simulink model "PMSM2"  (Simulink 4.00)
settings: Solver=ode23  StartTime=-eps  StopTime=2  FixedStep=0.000001  RelTol=1e-3
undefined symbols (not defined in the file or in its folder): J, Lsx, Lsy, p, Psim, Rs, sfunxy, Ts, Udc

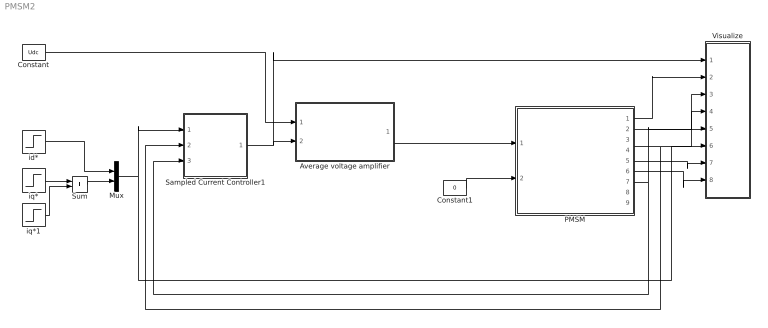
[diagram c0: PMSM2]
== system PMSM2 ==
  Average voltage amplifier : Subsystem
  Constant : Constant  Value=Udc
  Constant1 : Constant  Value=0
  Mux : Mux  Inputs=2
  PMSM : Subsystem  mask{Psim=Psim, p=p, Rs=Rs, isy=[0 1], psisy=[0 Lsy], isx=[0 1], psisx=[0 Lsx], J=J}
      mask prompts: p "Number of poles"; Rs "Stator resistance"; isy "y-axis current vector"; psisy "y-axis flux vector"; isx "x-axis current vector"; psisx "x-axis flux vector"; J "Inertia"
  Sampled Current Controller1 : Subsystem  mask{R=Rs, Lx=Lsx, Ly=Lsy, Kp=[(Lsx/Ts+Rs/2) (Lsy/Ts+Rs/2)]', Ti=[(Lsx/Rs+Ts/2) (Lsy/Rs+Ts/2)]', Ts=Ts, Umax=Udc, Umin=-Udc, SlowFast=Fast computer}
      mask prompts: R "Load resistance"; Lx "x-axis load inductance"; Ly "y-axis load inductance"; Kp "Controller gain"; Ti "Integral Time Constant"; Ts "Sampling time [s]"; Umax "Max output signal"; Umin "Min output signal"; SlowFast "Controller type"
  Sum : Sum  Inputs=++  SaturateOnIntegerOverflow=on
  Visualize : Subsystem
  id* : Step  Time=0.0105  Before=0  After=0  SampleTime=0
  iq* : Step  Time=0.0055  Before=0  After=10  SampleTime=0
  iq*1 : Step  Time=0.05  Before=0  After=0  SampleTime=0
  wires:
  Average voltage amplifier/1(vabc) -> PMSM/1(vabc)
  Sampled Current Controller1/1(u*) -> Visualize/1(u*), Average voltage amplifier/2(uabc*)
  Constant/1 -> Average voltage amplifier/1(Udc)
  id*/1 -> Mux/1
  Mux/1 -> Visualize/6(i*dq), Sampled Current Controller1/1(Ref_dq)
  PMSM/7(theta_el) -> Visualize/5(theta), Sampled Current Controller1/3(thetaR)
  Constant1/1 -> PMSM/2(Tl)
  PMSM/1(uabc) -> Visualize/2("u ")
  PMSM/4(is) -> Visualize/4(i), Sampled Current Controller1/2(Act_ab)
  PMSM/2(exy) -> Visualize/3(e)
  PMSM/5(T_mech) -> Visualize/7(Tmech)
  PMSM/6(w_mech) -> Visualize/8(wmech)
  iq*/1 -> Sum/1
  iq*1/1 -> Sum/2
  Sum/1 -> Mux/2

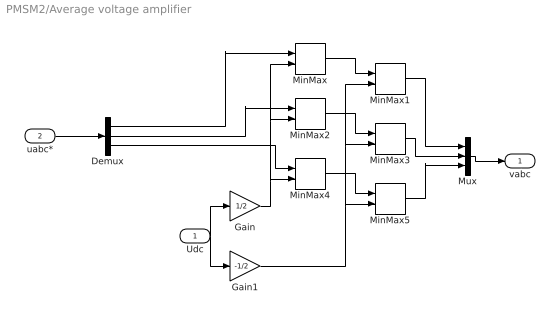
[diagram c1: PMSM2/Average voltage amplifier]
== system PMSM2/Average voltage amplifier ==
  Udc : Inport  Port=1  LatchInput=off
  uabc* : Inport  Port=2  LatchInput=off
  Demux : Demux  Outputs=3  BusSelectionMode=off
  Gain : Gain  Gain=1/2  Multiplication=Element-wise(K.*u)  SaturateOnIntegerOverflow=on
  Gain1 : Gain  Gain=-1/2  Multiplication=Element-wise(K.*u)  SaturateOnIntegerOverflow=on
  MinMax : MinMax  Function=min  Inputs=2
  MinMax1 : MinMax  Function=max  Inputs=2
  MinMax2 : MinMax  Function=min  Inputs=2
  MinMax3 : MinMax  Function=max  Inputs=2
  MinMax4 : MinMax  Function=min  Inputs=2
  MinMax5 : MinMax  Function=max  Inputs=2
  Mux : Mux  Inputs=3
  vabc : Outport  Port=1  InitialOutput=0
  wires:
  MinMax/1 -> MinMax1/1
  Udc/1 -> Gain/1, Gain1/1
  Gain/1 -> MinMax/2, MinMax2/2, MinMax4/2
  Gain1/1 -> MinMax1/2, MinMax3/2, MinMax5/2
  MinMax2/1 -> MinMax3/1
  MinMax4/1 -> MinMax5/1
  uabc*/1 -> Demux/1
  Demux/1 -> MinMax/1
  Demux/2 -> MinMax2/1
  Demux/3 -> MinMax4/1
  MinMax1/1 -> Mux/1
  MinMax3/1 -> Mux/2
  MinMax5/1 -> Mux/3
  Mux/1 -> vabc/1

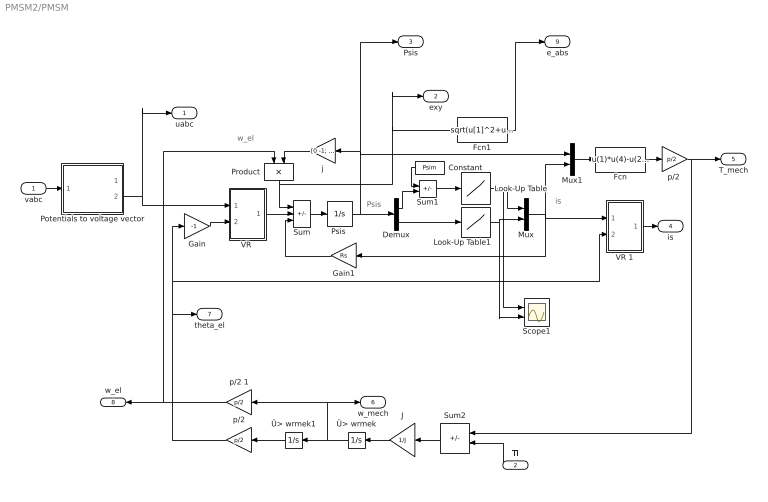
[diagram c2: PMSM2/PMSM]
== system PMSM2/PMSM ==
  note: w_el
  note: Psis
  note: is
  vabc : Inport  Port=1  LatchInput=off
  Tl : Inport  Orientation=left  Port=2  LatchInput=off
  Constant : Constant  Orientation=left  Value=Psim
  Demux : Demux  Outputs=2  BusSelectionMode=off
  Fcn : Fcn  Expr=u(1)*u(4)-u(2)*u(3)
  Fcn1 : Fcn  Expr=sqrt(u[1]^2+u[2]^2)
  Gain : Gain  Gain=-1  Multiplication=Element-wise(K.*u)  SaturateOnIntegerOverflow=on
  Gain1 : Gain  Orientation=left  Gain=Rs  Multiplication=Element-wise(K.*u)  SaturateOnIntegerOverflow=on
  J : Gain  Orientation=left  Gain=1/J  Multiplication=Element-wise(K.*u)  SaturateOnIntegerOverflow=on
  Look-Up Table : Lookup  InputValues=psisx  OutputValues=isx
  Look-Up Table1 : Lookup  InputValues=psisy  OutputValues=isy
  Mux : Mux  Inputs=2
  Mux1 : Mux  Inputs=2
  Potentials to voltage vector : Subsystem
  Product : Product  Orientation=down  Inputs=2  Multiplication=Element-wise(.*)  SaturateOnIntegerOverflow=on
  "Psis " : Integrator  ExternalReset=none  InitialConditionSource=internal  InitialCondition=[Psim 0]'  LimitOutput=on  UpperSaturationLimit=[2*Psim Psim*2]'  LowerSaturationLimit=[Psim/20 0]'  ShowSaturationPort=off  ShowStatePort=off  AbsoluteTolerance=auto
  Scope1 : Scope  NumInputPorts=2
  Sum : Sum  Inputs=-+-  SaturateOnIntegerOverflow=on
  Sum1 : Sum  Inputs=-+  SaturateOnIntegerOverflow=on
  Sum2 : Sum  Orientation=left  Inputs=+-  SaturateOnIntegerOverflow=on
  "VR " : Subsystem
  VR 1 : Subsystem
  j : Gain  Orientation=left  Gain=[0 -1; 1 0]  Multiplication=Matrix(K*u)  SaturateOnIntegerOverflow=on
  p/2 : Gain  Orientation=left  Gain=p/2  Multiplication=Matrix(K*u)  SaturateOnIntegerOverflow=on
  "p/2 " : Gain  Gain=p/2  Multiplication=Matrix(K*u)  SaturateOnIntegerOverflow=on
  p/2 1 : Gain  Orientation=left  Gain=p/2  Multiplication=Matrix(K*u)  SaturateOnIntegerOverflow=on
  Ü> wrmek : Integrator  Orientation=left  ExternalReset=none  InitialConditionSource=internal  InitialCondition=0  LimitOutput=off  UpperSaturationLimit=inf  LowerSaturationLimit=-inf  ShowSaturationPort=off  ShowStatePort=off  AbsoluteTolerance=auto
  Ü> wrmek1 : Integrator  Orientation=left  ExternalReset=none  InitialConditionSource=internal  InitialCondition=0  LimitOutput=off  UpperSaturationLimit=inf  LowerSaturationLimit=-inf  ShowSaturationPort=off  ShowStatePort=off  AbsoluteTolerance=auto
  uabc : Outport  Port=1
  exy : Outport  Port=2
  Psis : Outport  Port=3
  is : Outport  Port=4
  T_mech : Outport  Port=5
  w_mech : Outport  Port=6
  theta_el : Outport  Port=7
  w_el : Outport  Orientation=left  Port=8
  e_abs : Outport  Port=9
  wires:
  VR 1/1(Out) -> is/1
  Ü> wrmek/1 -> Ü> wrmek1/1, p/2 1/1, w_mech/1
  Fcn1/1 -> e_abs/1
  p/2 1/1 -> w_el/1, Product/1
  Tl/1 -> Sum2/2
  Ü> wrmek1/1 -> p/2/1
  Sum2/1 -> J/1
  J/1 -> Ü> wrmek/1
  vabc/1 -> Potentials to voltage vector/1(In1)
  Potentials to voltage vector/2(uab) -> "VR "/1(vect), uabc/1
  "p/2 "/1 -> Sum2/1, T_mech/1
  Gain/1 -> "VR "/2(angle)
  Sum/1 -> "Psis "/1
  "Psis "/1 -> Demux/1, j/1, Mux1/1, Psis/1
  Demux/1 -> Sum1/2
  Demux/2 -> Look-Up Table1/1
  Look-Up Table/1 -> Scope1/1, Mux/1
  Look-Up Table1/1 -> Scope1/2, Mux/2
  Mux/1 -> Mux1/2, Gain1/1, VR 1/1(vect)
  Mux1/1 -> Fcn/1
  Constant/1 -> Sum1/1
  Sum1/1 -> Look-Up Table/1
  Gain1/1 -> Sum/3
  "VR "/1(Out) -> Sum/2
  Product/1 -> Sum/1, Fcn1/1, exy/1
  Fcn/1 -> "p/2 "/1
  j/1 -> Product/2
  p/2/1 -> theta_el/1, Gain/1, VR 1/2(angle)

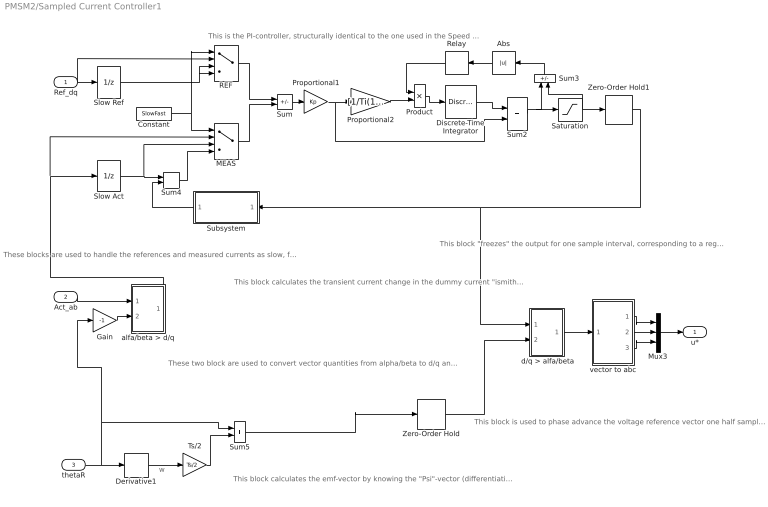
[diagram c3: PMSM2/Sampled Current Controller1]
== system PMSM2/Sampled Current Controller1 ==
  note: These blocks are used to handle the references and measured currents as slow, fast or fast computer with Smith predictor.
  note: This block calculates the transient current change in the dummy current "ismith" The smith predictor calculates the current change that would have been measured if the computer was "fast", i.e. without the delay that a slow computer has. The calculated current change equals the real current change, but informing the controller one sampling interval earlier, thus allowing a high (deadbeat) gain.
  note: This is the PI-controller, structurally identical to the one used in the Speed Controller
  note: This block "freezes" the output for one sample interval, corresponding to a register in a microcontroller where the reference voltages are written once every sampling inteval.
  note: These two block are used to convert vector quantities from alpha/beta to d/q and back again. Note that they are identical, but use the angle with opposite sign.
  note: This block calculates the emf-vector by knowing the "Psi"-vector (differentiation) and calculates the emf- components in the d/q-plane (ideally there is only "eq" whilse "ed"=0). It alse calculates the angle of the "Psi"- vector, used to orient the d/q-plane.
  note: This block is used to phase advance the voltage reference vector one half sample period. It is done to compensate for the fact that the "reality" is turning during the same sample period as the voltage references are being held constant. In the beginning of the sample period, the voltage reference will be 1/2 sample period ahead of reality, and in the end of the sample period it will be 1/2 period behind. In average, it will be in the correct position relative to reality.
  note: w
  Ref_dq : Inport  Port=1  LatchInput=off
  Act_ab : Inport  Port=2  LatchInput=off
  thetaR : Inport  Port=3  LatchInput=off
  " d/q > alfa/beta" : Subsystem
  Abs : Abs  Orientation=left  SaturateOnIntegerOverflow=on
  Constant : Constant  Value=SlowFast
  Derivative1 : Derivative
  Discrete-Time Integrator : DiscreteIntegrator  IntegratorMethod=ForwardEuler  ExternalReset=none  InitialConditionSource=internal  InitialCondition=0  LimitOutput=on  UpperSaturationLimit=Umax  LowerSaturationLimit=Umin  ShowSaturationPort=off  ShowStatePort=off  SampleTime=Ts
  Gain : Gain  Gain=-1  Multiplication=Element-wise(K.*u)  SaturateOnIntegerOverflow=on
  MEAS : MultiPortSwitch  Inputs=3
  Mux3 : Mux  Inputs=3
  Product : Product  Inputs=2  Multiplication=Element-wise(.*)  SaturateOnIntegerOverflow=on
  Proportional1 : Gain  Gain=Kp  Multiplication=Element-wise(K.*u)  SaturateOnIntegerOverflow=on
  Proportional2 : Gain  Gain=[1/Ti(1) 1/Ti(2)]  Multiplication=Element-wise(K.*u)  SaturateOnIntegerOverflow=on
  REF : MultiPortSwitch  Inputs=3
  Relay : Relay  Orientation=left  OnSwitchValue=eps  OffSwitchValue=eps  OnOutputValue=0  OffOutputValue=1
  Saturation : Saturate  UpperLimit=Umax  LowerLimit=Umin  LinearizeAsGain=on
  Slow Act : UnitDelay  X0=0  SampleTime=Ts
  Slow Ref : UnitDelay  X0=0  SampleTime=Ts
  Subsystem : Subsystem  Orientation=left
  Sum : Sum  Inputs=+-  SaturateOnIntegerOverflow=on
  Sum2 : Sum  Inputs=++  SaturateOnIntegerOverflow=on
  Sum3 : Sum  Orientation=up  Inputs=+-  SaturateOnIntegerOverflow=on
  Sum4 : Sum  Inputs=++  SaturateOnIntegerOverflow=on
  Sum5 : Sum  Inputs=++  SaturateOnIntegerOverflow=on
  Ts/2 : Gain  Gain=Ts/2  Multiplication=Matrix(K*u)  SaturateOnIntegerOverflow=on
  Zero-Order Hold : ZeroOrderHold  SampleTime=Ts
  Zero-Order Hold1 : ZeroOrderHold  SampleTime=Ts
  alfa/beta > d/q : Subsystem
  vector to abc : Subsystem
  u* : Outport  Port=1
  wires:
  Discrete-Time Integrator/1 -> Sum2/1
  Proportional1/1 -> Proportional2/1, Sum2/2
  Sum/1 -> Proportional1/1
  Sum2/1 -> Saturation/1, Sum3/1
  Saturation/1 -> Zero-Order Hold1/1, Sum3/2
  Proportional2/1 -> Product/2
  Product/1 -> Discrete-Time Integrator/1
  Relay/1 -> Product/1
  Ref_dq/1 -> REF/2, Slow Ref/1
  Zero-Order Hold1/1 -> Subsystem/1(u), " d/q > alfa/beta"/1(vect)
  Slow Act/1 -> Sum4/1, MEAS/3
  Subsystem/1(di_smith) -> Sum4/2
  Constant/1 -> MEAS/1, REF/1
  Slow Ref/1 -> REF/3, REF/4
  REF/1 -> Sum/1
  Sum4/1 -> MEAS/4
  MEAS/1 -> Sum/2
  Sum3/1 -> Abs/1
  Abs/1 -> Relay/1
  Gain/1 -> alfa/beta > d/q/2(angle)
  Act_ab/1 -> alfa/beta > d/q/1(vect)
  Sum5/1 -> Zero-Order Hold/1
  Zero-Order Hold/1 -> " d/q > alfa/beta"/2(angle)
  " d/q > alfa/beta"/1(Out) -> vector to abc/1(vect)
  vector to abc/1(a) -> Mux3/1
  vector to abc/2(b) -> Mux3/2
  vector to abc/3(c) -> Mux3/3
  alfa/beta > d/q/1(Out) -> Slow Act/1, MEAS/2
  Mux3/1 -> u*/1
  thetaR/1 -> Derivative1/1, Gain/1, Sum5/1
  Derivative1/1 -> Ts/2/1
  Ts/2/1 -> Sum5/2

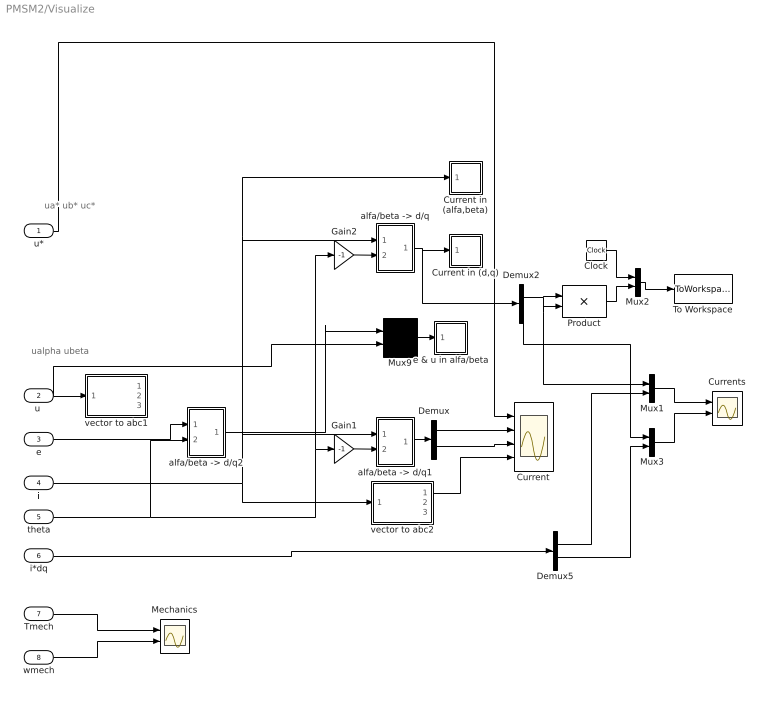
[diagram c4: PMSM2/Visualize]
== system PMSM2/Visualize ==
  note: ua* ub* uc*
  note: ualpha ubeta
  u* : Inport  Port=1  LatchInput=off
  "u " : Inport  Port=2  LatchInput=off
  e : Inport  Port=3  LatchInput=off
  i : Inport  Port=4  LatchInput=off
  theta : Inport  Port=5  LatchInput=off
  i*dq : Inport  Port=6  LatchInput=off
  Tmech : Inport  Port=7  LatchInput=off
  wmech : Inport  Port=8  LatchInput=off
  Clock : Clock
  Current : Scope  NumInputPorts=4
  Current in (alfa,beta) : Subsystem  LoadFcn=sfunxy([],[],[],'LoadBlock')  StartFcn=sfunxy([],[],[],'Start')  StopFcn=sfunxy([],[],[],'Stop')  mask(XY scope.){xmin=-20, xmax=20, ymin=-20, ymax=20, st=-1}
      mask prompts: xmin "x-min:"; xmax "x-max:"; ymin "y-min:"; ymax "y-max:"; st "Sample time:"
      mask help: XY scope using MATLAB graph window. First input is used as time base. Enter plotting ranges.
  Current in (d,q) : Subsystem  LoadFcn=sfunxy([],[],[],'LoadBlock')  StartFcn=sfunxy([],[],[],'Start')  StopFcn=sfunxy([],[],[],'Stop')  mask(XY scope.){xmin=-20, xmax=20, ymin=-20, ymax=20, st=-1}
      mask prompts: xmin "x-min:"; xmax "x-max:"; ymin "y-min:"; ymax "y-max:"; st "Sample time:"
      mask help: XY scope using MATLAB graph window. First input is used as time base. Enter plotting ranges.
  Currents : Scope  NumInputPorts=2
  Demux : Demux  Outputs=2  BusSelectionMode=off
  Demux2 : Demux  Outputs=2  BusSelectionMode=off
  Demux5 : Demux  Outputs=2  BusSelectionMode=off
  Gain1 : Gain  Gain=-1  Multiplication=Element-wise(K.*u)  SaturateOnIntegerOverflow=on
  Gain2 : Gain  Gain=-1  Multiplication=Element-wise(K.*u)  SaturateOnIntegerOverflow=on
  Mechanics : Scope  NumInputPorts=2
  Mux{1..3,9} (4 alike) : Mux  Inputs=2
  Product : Product  Inputs=2  Multiplication=Element-wise(.*)  SaturateOnIntegerOverflow=on
  To Workspace : ToWorkspace  VariableName=f1  SampleTime=-1  SaveFormat=Array
  "alfa/beta -> d/q" : Subsystem
  "alfa/beta -> d/q1" : Subsystem
  "alfa/beta -> d/q2" : Subsystem
  e & u in alfa/beta : Subsystem  LoadFcn=sfunxy([],[],[],'LoadBlock')  StartFcn=sfunxy([],[],[],'Start')  StopFcn=sfunxy([],[],[],'Stop')  mask(XY scope.){xmin=-300, xmax=300, ymin=-300, ymax=300, st=-1}
      mask prompts: xmin "x-min:"; xmax "x-max:"; ymin "y-min:"; ymax "y-max:"; st "Sample time:"
      mask help: XY scope using MATLAB graph window. First input is used as time base. Enter plotting ranges.
  vector to abc1 : Subsystem
  vector to abc2 : Subsystem
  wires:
  Gain2/1 -> "alfa/beta -> d/q"/2(angle)
  Gain1/1 -> "alfa/beta -> d/q1"/2(angle)
  "alfa/beta -> d/q1"/1(Out) -> Demux/1
  Demux/1 -> Current/2
  Demux/2 -> Current/3
  vector to abc2/1(a) -> Current/4
  "alfa/beta -> d/q"/1(Out) -> Current in (d,q)/1(xy), Demux2/1
  u*/1 -> Current/1
  "u "/1 -> vector to abc1/1(vect), Mux9/2
  i/1 -> Current in (alfa,beta)/1(xy), "alfa/beta -> d/q"/1(vect), "alfa/beta -> d/q1"/1(vect), vector to abc2/1(vect)
  Mux9/1 -> e & u in alfa/beta/1(xy)
  theta/1 -> Gain1/1, Gain2/1, "alfa/beta -> d/q2"/2(angle)
  Clock/1 -> Mux2/1
  Product/1 -> Mux2/2
  Mux2/1 -> To Workspace/1
  Demux2/1 -> Product/1, Product/2, Mux1/1
  i*dq/1 -> Demux5/1
  Demux5/1 -> Mux1/2
  Demux2/2 -> Mux3/1
  Demux5/2 -> Mux3/2
  Mux3/1 -> Currents/2
  Mux1/1 -> Currents/1
  e/1 -> "alfa/beta -> d/q2"/1(vect)
  "alfa/beta -> d/q2"/1(Out) -> Mux9/1
  Tmech/1 -> Mechanics/1
  wmech/1 -> Mechanics/2

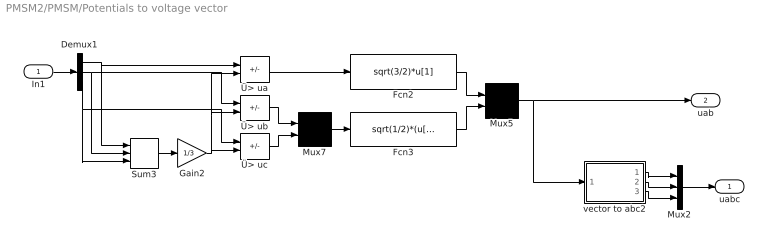
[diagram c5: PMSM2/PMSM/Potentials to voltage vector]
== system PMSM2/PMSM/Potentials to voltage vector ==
  In1 : Inport  Port=1  LatchInput=off
  Demux1 : Demux  Outputs=3  BusSelectionMode=off
  Fcn2 : Fcn  Expr=sqrt(3/2)*u[1]
  Fcn3 : Fcn  Expr=sqrt(1/2)*(u[1]-u[2])
  Gain2 : Gain  Gain=1/3  Multiplication=Element-wise(K.*u)  SaturateOnIntegerOverflow=on
  Mux2 : Mux  Inputs=3
  Mux5 : Mux  Inputs=2
  Mux7 : Mux  Inputs=2
  Sum3 : Sum  Inputs=+++  SaturateOnIntegerOverflow=on
  vector to abc2 : Subsystem
  Ü> ua : Sum  Inputs=+-  SaturateOnIntegerOverflow=on
  Ü> ub : Sum  Inputs=+-  SaturateOnIntegerOverflow=on
  Ü> uc : Sum  Inputs=+-  SaturateOnIntegerOverflow=on
  uabc : Outport  Port=1
  uab : Outport  Port=2
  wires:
  Fcn3/1 -> Mux5/2
  Fcn2/1 -> Mux5/1
  Mux7/1 -> Fcn3/1
  Ü> uc/1 -> Mux7/2
  Ü> ub/1 -> Mux7/1
  Ü> ua/1 -> Fcn2/1
  Gain2/1 -> Ü> uc/2, Ü> ub/2, Ü> ua/2
  Demux1/2 -> Ü> ub/1, Sum3/2
  Sum3/1 -> Gain2/1
  Demux1/3 -> Ü> uc/1, Sum3/3
  Demux1/1 -> Ü> ua/1, Sum3/1
  In1/1 -> Demux1/1
  Mux5/1 -> uab/1, vector to abc2/1(vect)
  vector to abc2/1(a) -> Mux2/1
  vector to abc2/2(b) -> Mux2/2
  vector to abc2/3(c) -> Mux2/3
  Mux2/1 -> uabc/1

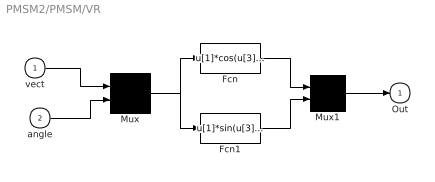
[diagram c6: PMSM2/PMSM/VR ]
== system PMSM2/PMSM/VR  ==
  vect : Inport  Port=1  LatchInput=off
  angle : Inport  Port=2  LatchInput=off
  Fcn : Fcn  Expr=u[1]*cos(u[3])-u[2]*sin(u[3])
  Fcn1 : Fcn  Expr=u[1]*sin(u[3])+u[2]*cos(u[3])
  Mux : Mux  Inputs=2
  Mux1 : Mux  Inputs=2
  Out : Outport  Port=1  InitialOutput=0
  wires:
  Mux1/1 -> Out/1
  Fcn1/1 -> Mux1/2
  Fcn/1 -> Mux1/1
  Mux/1 -> Fcn1/1, Fcn/1
  angle/1 -> Mux/2
  vect/1 -> Mux/1

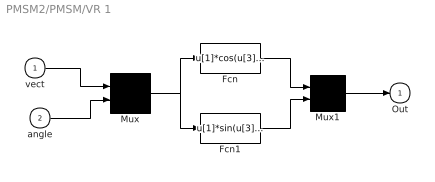
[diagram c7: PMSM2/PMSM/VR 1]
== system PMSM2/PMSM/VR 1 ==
  vect : Inport  Port=1  LatchInput=off
  angle : Inport  Port=2  LatchInput=off
  Fcn : Fcn  Expr=u[1]*cos(u[3])-u[2]*sin(u[3])
  Fcn1 : Fcn  Expr=u[1]*sin(u[3])+u[2]*cos(u[3])
  Mux : Mux  Inputs=2
  Mux1 : Mux  Inputs=2
  Out : Outport  Port=1  InitialOutput=0
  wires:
  vect/1 -> Mux/1
  angle/1 -> Mux/2
  Mux/1 -> Fcn/1, Fcn1/1
  Fcn/1 -> Mux1/1
  Fcn1/1 -> Mux1/2
  Mux1/1 -> Out/1

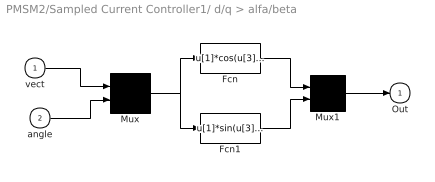
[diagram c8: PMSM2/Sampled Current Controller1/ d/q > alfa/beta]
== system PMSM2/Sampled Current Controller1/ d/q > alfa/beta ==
  vect : Inport  Port=1  LatchInput=off
  angle : Inport  Port=2  LatchInput=off
  Fcn : Fcn  Expr=u[1]*cos(u[3])-u[2]*sin(u[3])
  Fcn1 : Fcn  Expr=u[1]*sin(u[3])+u[2]*cos(u[3])
  Mux : Mux  Inputs=2
  Mux1 : Mux  Inputs=2
  Out : Outport  Port=1  InitialOutput=0
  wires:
  Mux1/1 -> Out/1
  Fcn1/1 -> Mux1/2
  Fcn/1 -> Mux1/1
  Mux/1 -> Fcn1/1, Fcn/1
  angle/1 -> Mux/2
  vect/1 -> Mux/1

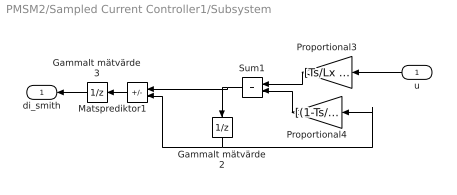
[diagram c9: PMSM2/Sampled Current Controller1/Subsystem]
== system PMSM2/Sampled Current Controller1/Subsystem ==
  u : Inport  Orientation=left  Port=1  LatchInput=off
  Gammalt mätvärde2 : UnitDelay  Orientation=down  X0=0  SampleTime=Ts
  Gammalt mätvärde3 : UnitDelay  Orientation=left  X0=0  SampleTime=Ts
  Matsprediktor1 : Sum  Orientation=left  Inputs=+-  SaturateOnIntegerOverflow=on
  Proportional3 : Gain  Orientation=left  Gain=[Ts/Lx Ts/Ly]  Multiplication=Element-wise(K.*u)  SaturateOnIntegerOverflow=on
  Proportional4 : Gain  Orientation=left  Gain=[(1-Ts/(Lx/R)) (1-Ts/(Ly/R))]  Multiplication=Element-wise(K.*u)  SaturateOnIntegerOverflow=on
  Sum1 : Sum  Orientation=left  Inputs=++  SaturateOnIntegerOverflow=on
  di_smith : Outport  Orientation=left  Port=1
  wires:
  Proportional3/1 -> Sum1/1
  Proportional4/1 -> Sum1/2
  Sum1/1 -> Gammalt mätvärde2/1, Matsprediktor1/1
  u/1 -> Proportional3/1
  Matsprediktor1/1 -> Gammalt mätvärde3/1
  Gammalt mätvärde3/1 -> di_smith/1
  Gammalt mätvärde2/1 -> Proportional4/1, Matsprediktor1/2

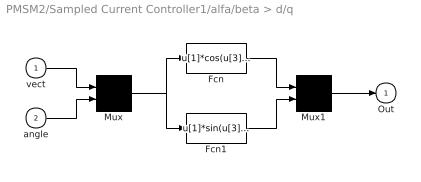
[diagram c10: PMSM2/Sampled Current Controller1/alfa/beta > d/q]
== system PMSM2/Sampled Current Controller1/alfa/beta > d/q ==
  vect : Inport  Port=1  LatchInput=off
  angle : Inport  Port=2  LatchInput=off
  Fcn : Fcn  Expr=u[1]*cos(u[3])-u[2]*sin(u[3])
  Fcn1 : Fcn  Expr=u[1]*sin(u[3])+u[2]*cos(u[3])
  Mux : Mux  Inputs=2
  Mux1 : Mux  Inputs=2
  Out : Outport  Port=1  InitialOutput=0
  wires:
  vect/1 -> Mux/1
  angle/1 -> Mux/2
  Mux/1 -> Fcn/1, Fcn1/1
  Fcn/1 -> Mux1/1
  Fcn1/1 -> Mux1/2
  Mux1/1 -> Out/1

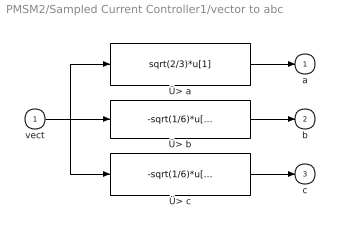
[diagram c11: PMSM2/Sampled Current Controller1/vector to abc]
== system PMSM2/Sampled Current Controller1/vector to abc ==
  vect : Inport  Port=1  LatchInput=off
  Ü> a : Fcn  Expr=sqrt(2/3)*u[1]
  Ü> b : Fcn  Expr=-sqrt(1/6)*u[1]+sqrt(1/2)*u[2]
  Ü> c : Fcn  Expr=-sqrt(1/6)*u[1]-sqrt(1/2)*u[2]
  a : Outport  Port=1  InitialOutput=0
  b : Outport  Port=2  InitialOutput=0
  c : Outport  Port=3  InitialOutput=0
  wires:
  vect/1 -> Ü> b/1, Ü> a/1, Ü> c/1
  Ü> b/1 -> b/1
  Ü> c/1 -> c/1
  Ü> a/1 -> a/1

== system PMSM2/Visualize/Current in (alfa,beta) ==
  xy : Inport  Port=1  LatchInput=off
  sfunxy : S-Function  FunctionName=sfunxy  Parameters=[xmin xmax ymin ymax], st  PortCounts=[]  SFunctionModules=''
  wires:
  xy/1 -> sfunxy/1

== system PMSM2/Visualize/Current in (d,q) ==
  xy : Inport  Port=1  LatchInput=off
  sfunxy : S-Function  FunctionName=sfunxy  Parameters=[xmin xmax ymin ymax], st  PortCounts=[]  SFunctionModules=''
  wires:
  xy/1 -> sfunxy/1

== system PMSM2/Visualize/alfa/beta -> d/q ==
  vect : Inport  Port=1  LatchInput=off
  angle : Inport  Port=2  LatchInput=off
  Fcn : Fcn  Expr=u[1]*cos(u[3])-u[2]*sin(u[3])
  Fcn1 : Fcn  Expr=u[1]*sin(u[3])+u[2]*cos(u[3])
  Mux : Mux  Inputs=2
  Mux1 : Mux  Inputs=2
  Out : Outport  Port=1  InitialOutput=0
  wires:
  vect/1 -> Mux/1
  angle/1 -> Mux/2
  Mux/1 -> Fcn/1, Fcn1/1
  Fcn/1 -> Mux1/1
  Fcn1/1 -> Mux1/2
  Mux1/1 -> Out/1

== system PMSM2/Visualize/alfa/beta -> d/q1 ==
  vect : Inport  Port=1  LatchInput=off
  angle : Inport  Port=2  LatchInput=off
  Fcn : Fcn  Expr=u[1]*cos(u[3])-u[2]*sin(u[3])
  Fcn1 : Fcn  Expr=u[1]*sin(u[3])+u[2]*cos(u[3])
  Mux : Mux  Inputs=2
  Mux1 : Mux  Inputs=2
  Out : Outport  Port=1  InitialOutput=0
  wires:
  Mux1/1 -> Out/1
  Fcn1/1 -> Mux1/2
  Fcn/1 -> Mux1/1
  Mux/1 -> Fcn1/1, Fcn/1
  angle/1 -> Mux/2
  vect/1 -> Mux/1

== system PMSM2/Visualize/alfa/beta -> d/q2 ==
  vect : Inport  Port=1  LatchInput=off
  angle : Inport  Port=2  LatchInput=off
  Fcn : Fcn  Expr=u[1]*cos(u[3])-u[2]*sin(u[3])
  Fcn1 : Fcn  Expr=u[1]*sin(u[3])+u[2]*cos(u[3])
  Mux : Mux  Inputs=2
  Mux1 : Mux  Inputs=2
  Out : Outport  Port=1  InitialOutput=0
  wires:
  vect/1 -> Mux/1
  angle/1 -> Mux/2
  Mux/1 -> Fcn/1, Fcn1/1
  Fcn/1 -> Mux1/1
  Fcn1/1 -> Mux1/2
  Mux1/1 -> Out/1

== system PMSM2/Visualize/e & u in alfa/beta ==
  xy : Inport  Port=1  LatchInput=off
  sfunxy : S-Function  FunctionName=sfunxy4  Parameters=[xmin xmax ymin ymax], st  PortCounts=[]  SFunctionModules=''
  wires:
  xy/1 -> sfunxy/1

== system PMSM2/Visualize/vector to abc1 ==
  vect : Inport  Port=1  LatchInput=off
  Ü> a : Fcn  Expr=sqrt(2/3)*u[1]
  Ü> b : Fcn  Expr=-sqrt(1/6)*u[1]+sqrt(1/2)*u[2]
  Ü> c : Fcn  Expr=-sqrt(1/6)*u[1]-sqrt(1/2)*u[2]
  a : Outport  Port=1  InitialOutput=0
  b : Outport  Port=2  InitialOutput=0
  c : Outport  Port=3  InitialOutput=0
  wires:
  Ü> a/1 -> a/1
  Ü> c/1 -> c/1
  Ü> b/1 -> b/1
  vect/1 -> Ü> c/1, Ü> a/1, Ü> b/1

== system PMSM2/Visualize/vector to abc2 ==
  vect : Inport  Port=1  LatchInput=off
  Ü> a : Fcn  Expr=sqrt(2/3)*u[1]
  Ü> b : Fcn  Expr=-sqrt(1/6)*u[1]+sqrt(1/2)*u[2]
  Ü> c : Fcn  Expr=-sqrt(1/6)*u[1]-sqrt(1/2)*u[2]
  a : Outport  Port=1  InitialOutput=0
  b : Outport  Port=2  InitialOutput=0
  c : Outport  Port=3  InitialOutput=0
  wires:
  vect/1 -> Ü> b/1, Ü> a/1, Ü> c/1
  Ü> b/1 -> b/1
  Ü> c/1 -> c/1
  Ü> a/1 -> a/1

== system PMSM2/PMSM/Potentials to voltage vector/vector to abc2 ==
  vect : Inport  Port=1  LatchInput=off
  Ü> a : Fcn  Expr=sqrt(2/3)*u[1]
  Ü> b : Fcn  Expr=-sqrt(1/6)*u[1]+sqrt(1/2)*u[2]
  Ü> c : Fcn  Expr=-sqrt(1/6)*u[1]-sqrt(1/2)*u[2]
  a : Outport  Port=1  InitialOutput=0
  b : Outport  Port=2  InitialOutput=0
  c : Outport  Port=3  InitialOutput=0
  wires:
  vect/1 -> Ü> b/1, Ü> a/1, Ü> c/1
  Ü> b/1 -> b/1
  Ü> c/1 -> c/1
  Ü> a/1 -> a/1
